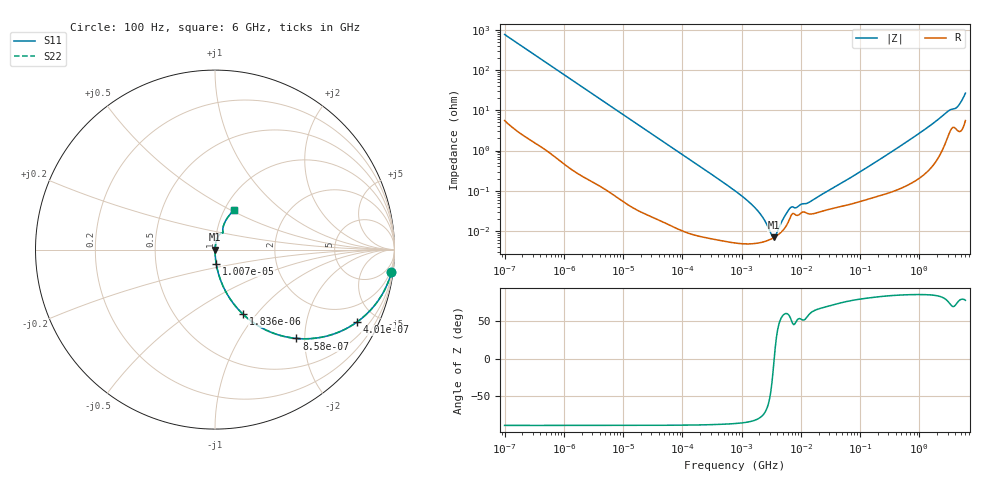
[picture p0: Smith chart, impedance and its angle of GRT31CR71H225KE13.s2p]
!Murata Part Number: GRT31CR71H225KE13
!These Parameters are Measured in Series Mode Connection
!Data Generated on Jun 19, 2026
!  o--ll--o
!Port1  Port2
!  o------o
!Operation Temp=25[degC], DC Bias Voltage=0[V]
!Freq. Start=100[Hz] Stop=6[GHz] 401[Steps]
# Hz S RI R 50
!Freq.(Hz) S11(Real) S11(Imag) S21(Real) S21(Imag) S12(Real) S12(Imag) S22(Real) S22(Imag)
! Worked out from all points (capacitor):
!   401 points, 100 Hz to 6 GHz, reference 50 ohm
!   read as one part in series: C = 2.05 uF near 109 Hz
!   lowest |Z| = 6.87 mohm at 3.55 MHz (marker M1)
!   series resonance near 3.555 MHz, so ESL is about 980 pH
!   S11 on the Smith chart (normalised r, x): 100 Hz: 1, -15; 401 Hz: 1.03, -3.88; 858 Hz: 1.01, -1.82; 1.836 kHz: 1.01, -0.85; 10.07 kHz: 1.00, -0.16; 6 GHz: 1.11, +0.52
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100  0.9827 -0.1267  0.0173 0.1267  0.0173 0.1267  0.9827 -0.1267
224  0.9218 -0.2653  0.0782 0.2653  0.0782 0.2653  0.9218 -0.2653
401  0.7889 -0.4048  0.2111 0.4048  0.2111 0.4048  0.7889 -0.4048
858  0.4534 -0.4948  0.5466 0.4948  0.5466 0.4948  0.4534 -0.4948
1836  0.1552 -0.3592  0.8448 0.3592  0.8448 0.3592  0.1552 -0.3592
2008  0.1334 -0.337  0.8666 0.337  0.8666 0.337  0.1334 -0.337
3759  0.043 -0.1995  0.957 0.1995  0.957 0.1995  0.043 -0.1995
10066  0.00661 -0.0777  0.9934 0.0777  0.9934 0.0777  0.00661 -0.0777
40335  0.00057 -0.0196  0.9994 0.0196  0.9994 0.0196  0.00057 -0.0196
774597  5.07e-05 -0.000991  0.9999 0.000991  0.9999 0.000991  5.07e-05 -0.000991
1658239  4.83e-05 -0.000382  1 0.000382  1 0.000382  4.83e-05 -0.000382
2169299  5.16e-05 -0.000235  0.9999 0.000235  0.9999 0.000235  5.16e-05 -0.000235
2967816  6.01e-05 -8.32e-05  0.9999 8.32e-05  0.9999 8.32e-05  6.01e-05 -8.32e-05
3549919  6.87e-05 -6e-07  0.9999 6e-07  0.9999 6e-07  6.87e-05 -6e-07
4246196  8.22e-05 8.31e-05  0.9999 -8.31e-05  0.9999 -8.31e-05  8.22e-05 8.31e-05
5554849  0.000126 0.000221  0.9999 -0.000221  0.9999 -0.000221  0.000126 0.000221
6644369  0.000217 0.000305  0.9998 -0.000305  0.9998 -0.000305  0.000217 0.000305
1.555665e7  0.000264 0.000509  0.9997 -0.000509  0.9997 -0.000509  0.000264 0.000509
3.124326e8  0.000958 0.00849  0.999 -0.00849  0.999 -0.00849  0.000958 0.00849
3.065283e9  0.0302 0.0879  0.9698 -0.0879  0.9698 -0.0879  0.0302 0.0879
4.193612e9  0.0437 0.1016  0.9563 -0.1016  0.9563 -0.1016  0.0437 0.1016
6e9  0.1076 0.2213  0.8924 -0.2213  0.8924 -0.2213  0.1076 0.2213
